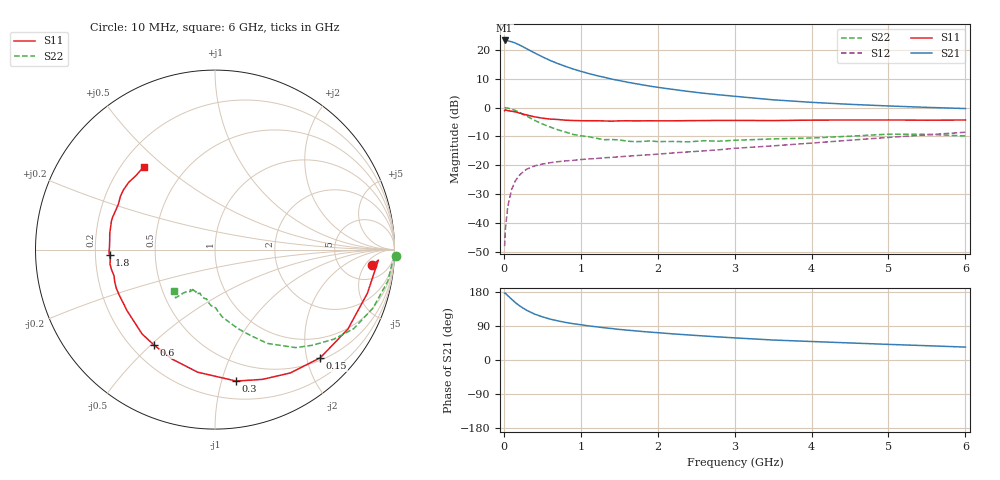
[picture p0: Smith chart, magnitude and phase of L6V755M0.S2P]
!  INFINEON TECHNOLOGIES Small Signal Semiconductors
! BFR380L3 , Si-NPN RF-Transistor in TSLP-3-1
!  Vce=0.75 V,  Ic=5 mA
! Common Emitter S-Parameters:  07. March 2005
#  GHz  S  MA  R  50
! f  S11  S21  S12  S22
! GHz  Mag  Ang  Mag  Ang  Mag  Ang  Mag  Ang
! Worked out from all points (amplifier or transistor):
!   36 points, 10 MHz to 6 GHz, reference 50 ohm
!   highest |S21| = 23.2 dB at 10 MHz (marker M1)
!   |S21| within 3 dB of that: start of sweep to 305.7 MHz
!   unconditionally stable (mu >= 1): 2.284 GHz to 4.967 GHz
!   at 250 MHz: K = 0.18, MSG = 21.6 dB, |S12| = -22.2 dB
!   at 1.4 GHz: K = 0.79, MSG = 13.6 dB, |S12| = -17.3 dB
!   at 6 GHz: K = 0.98, MSG = 4.1 dB, |S12| = -8.6 dB
!   S11 on the Smith chart (normalised r, x): 10 MHz: 10, -8; 150 MHz: 0.55, -2.26; 300 MHz: 0.34, -1.12; 600 MHz: 0.29, -0.51; 1.8 GHz: 0.26, -0.03; 6 GHz: 0.29, +0.42
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0.01  0.8803 -5.6  14.45 176.4  0.004 87.2  1.008 -2.1
0.02  0.912 -3.7  14.43 176.4  0.0078 89.7  0.9902 -4.4
0.05  0.8834 -15.9  14.26 170.0  0.0191 83.0  0.9785 -10.4
0.1  0.8628 -30.9  13.72 160.6  0.0379 74.3  0.9386 -20.3
0.15  0.8409 -45.8  13.03 151.6  0.0541 66.9  0.8896 -29.7
0.2  0.8052 -58.6  12.12 143.6  0.0666 61.4  0.8292 -37.0
0.25  0.7699 -69.9  11.21 137.0  0.0772 56.0  0.7614 -44.4
0.3  0.742 -80.8  10.32 130.8  0.0861 51.6  0.7078 -50.5
0.4  0.6899 -98.0  8.798 121.1  0.0978 45.5  0.5997 -60.7
0.5  0.6553 -111.4  7.545 114.0  0.1051 41.8  0.52 -67.3
0.6  0.6314 -122.5  6.528 108.0  0.111 39.6  0.4609 -73.5
0.7  0.6211 -130.9  5.77 103.4  0.1155 38.3  0.4132 -78.8
0.8  0.6031 -138.6  5.15 99.3  0.1194 37.6  0.3769 -83.9
1.1  0.5907 -154.5  3.88 90.1  0.1291 37.7  0.3138 -93.8
1.4  0.5811 -165.3  3.109 83.1  0.137 39.2  0.2794 -100.9
1.8  0.588 -176.9  2.47 75.2  0.15 42.2  0.2584 -109.4
2.2  0.5889 175.1  2.055 68.9  0.1638 45.3  0.2588 -114.1
2.8  0.5984 164.7  1.657 60.8  0.1861 49.8  0.2618 -121.6
3.5  0.5944 155.1  1.359 52.7  0.2172 52.4  0.2862 -124.4
4.5  0.609 146.9  1.135 45.0  0.2721 55.9  0.3194 -127.6
5.5  0.6032 137.0  1.006 37.7  0.3371 55.6  0.3431 -131.3
6  0.6083 130.9  0.96 34.1  0.3734 54.4  0.3229 -135.0
